FUNCTION_BLOCK Program_Assembled_Move_DUT

VAR_IN_OUT
    SD_SMD_IO: DUT_AMCI_Stepper;
END_VAR	

VAR_INPUT
	FB_Number_of_Segments: WORD; 
	
    FB_Segment_1_Distance: DINT;
    FB_Segment_1_Programmed_Speed: UDINT;
	FB_Segment_1_Acceleration: UINT;
	FB_Segment_1_Deceleration: UINT;
	
	FB_Segment_2_Distance: DINT;
    FB_Segment_2_Programmed_Speed: UDINT;
	FB_Segment_2_Acceleration: UINT;
	FB_Segment_2_Deceleration: UINT;
	
	FB_Segment_3_Distance: DINT;
    FB_Segment_3_Programmed_Speed: UDINT;
	FB_Segment_3_Acceleration: UINT;
	FB_Segment_3_Deceleration: UINT;
	
	FB_Segment_4_Distance: DINT;
    FB_Segment_4_Programmed_Speed: UDINT;
	FB_Segment_4_Acceleration: UINT;
	FB_Segment_4_Deceleration: UINT;
	
	FB_Segment_5_Distance: DINT;
    FB_Segment_5_Programmed_Speed: UDINT;
	FB_Segment_5_Acceleration: UINT;
	FB_Segment_5_Deceleration: UINT;
	
	FB_Segment_6_Distance: DINT;
    FB_Segment_6_Programmed_Speed: UDINT;
	FB_Segment_6_Acceleration: UINT;
	FB_Segment_6_Deceleration: UINT;
	
	FB_Segment_7_Distance: DINT;
    FB_Segment_7_Programmed_Speed: UDINT;
	FB_Segment_7_Acceleration: UINT;
	FB_Segment_7_Deceleration: UINT;
	
	FB_Segment_8_Distance: DINT;
    FB_Segment_8_Programmed_Speed: UDINT;
	FB_Segment_8_Acceleration: UINT;
	FB_Segment_8_Deceleration: UINT;
	
	FB_Segment_9_Distance: DINT;
    FB_Segment_9_Programmed_Speed: UDINT;
	FB_Segment_9_Acceleration: UINT;
	FB_Segment_9_Deceleration: UINT;
	
	FB_Segment_10_Distance: DINT;
    FB_Segment_10_Programmed_Speed: UDINT;
	FB_Segment_10_Acceleration: UINT;
	FB_Segment_10_Deceleration: UINT;
	
	FB_Segment_11_Distance: DINT;
    FB_Segment_11_Programmed_Speed: UDINT;
	FB_Segment_11_Acceleration: UINT;
	FB_Segment_11_Deceleration: UINT;
	
	FB_Segment_12_Distance: DINT;
    FB_Segment_12_Programmed_Speed: UDINT;
	FB_Segment_12_Acceleration: UINT;
	FB_Segment_12_Deceleration: UINT;
	
	FB_Segment_13_Distance: DINT;
    FB_Segment_13_Programmed_Speed: UDINT;
	FB_Segment_13_Acceleration: UINT;
	FB_Segment_13_Deceleration: UINT;
	
	FB_Segment_14_Distance: DINT;
    FB_Segment_14_Programmed_Speed: UDINT;
	FB_Segment_14_Acceleration: UINT;
	FB_Segment_14_Deceleration: UINT;
	
	FB_Segment_15_Distance: DINT;
    FB_Segment_15_Programmed_Speed: UDINT;
	FB_Segment_15_Acceleration: UINT;
	FB_Segment_15_Deceleration: UINT;
	
	FB_Segment_16_Distance: DINT;
    FB_Segment_16_Programmed_Speed: UDINT;
	FB_Segment_16_Acceleration: UINT;
	FB_Segment_16_Deceleration: UINT;
	
END_VAR

VAR_OUTPUT
	Enable: BOOL :=FALSE;
	Error: BOOL :=TRUE;
	Assembled_Move_Programmed: BOOL;
	
END_VAR

VAR	
	I_Command_Word_1: UINT;
	Assembled_Move_counter: ctu;
	Assembled_Move_counter_CV: DINT;
	Assembled_move_counter_PV: WORD;
	Assembled_Move_counter_DN: BOOL;
	Assembled_move_counter_reset: BOOL;
	
	
	
END_VAR
VAR // added by the converter: edge detectors and wires of the graphical bodies
    _w1, _w2, _w3, _w4, _w5, _w6, _w7, _w8, _w9, _w10, _w11, _w12, _w13, _w14, _w15, _w16, _w17, _w18, _w19 : BOOL;
END_VAR

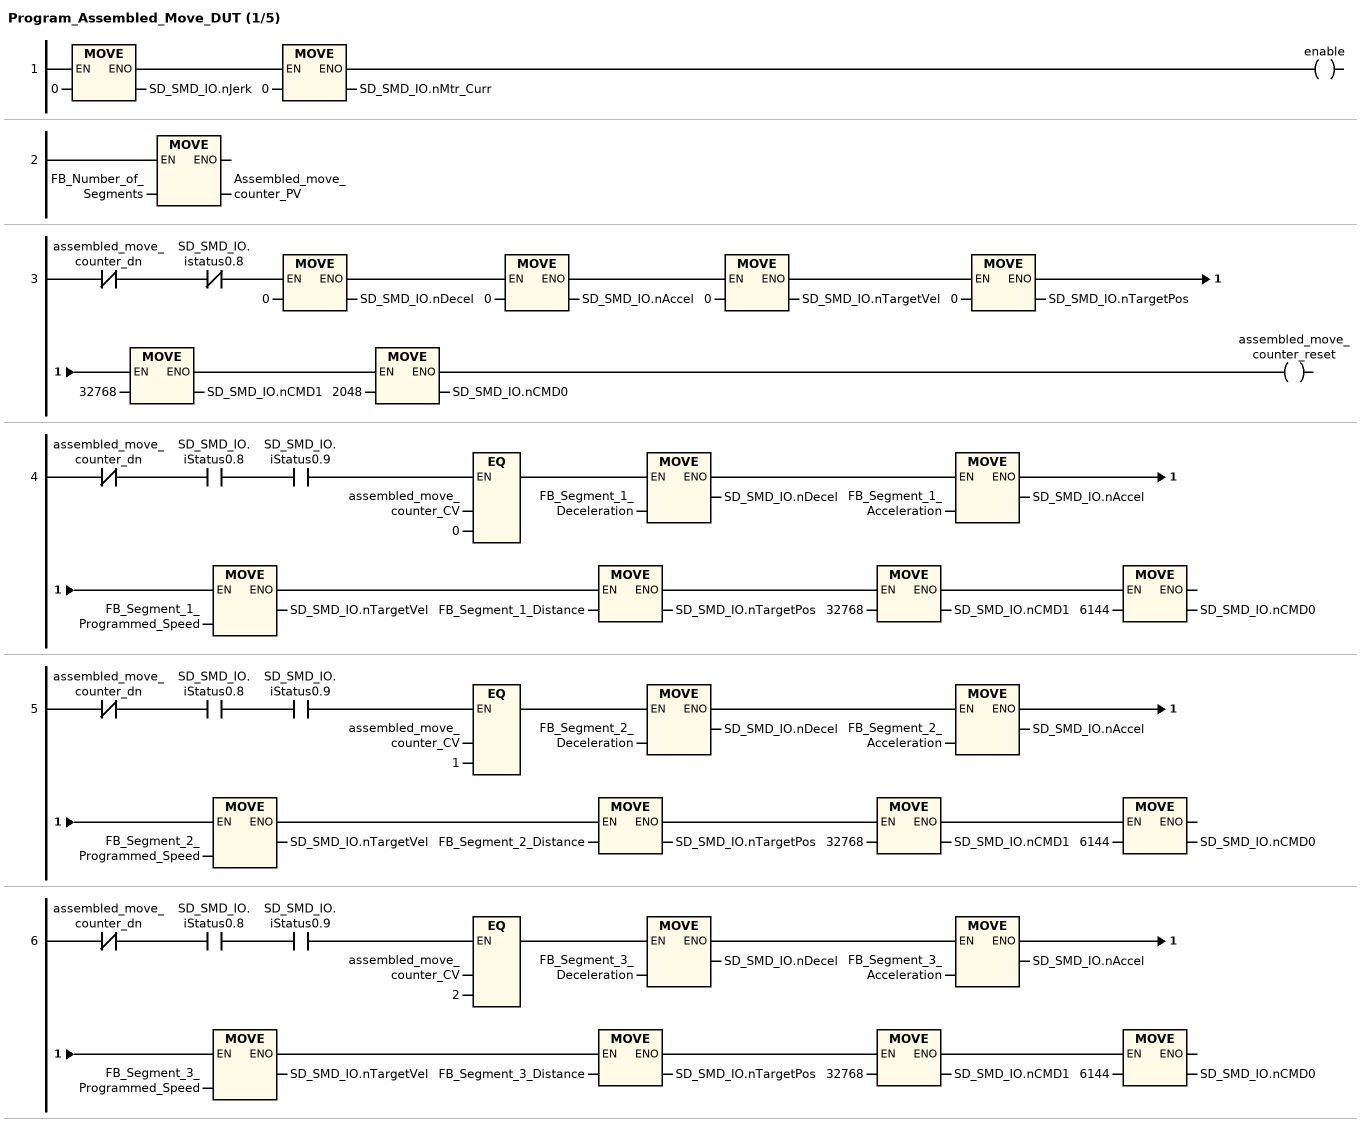
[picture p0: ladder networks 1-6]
// NETWORK 1
SD_SMD_IO.nJerk := 0;
SD_SMD_IO.nMtr_Curr := 0;
enable := TRUE;

// NETWORK 2
Assembled_move_counter_PV := FB_Number_of_Segments;

// NETWORK 3
_w1 := NOT assembled_move_counter_dn AND NOT SD_SMD_IO.istatus0.8;
IF _w1 THEN SD_SMD_IO.nDecel := 0; END_IF
IF _w1 THEN SD_SMD_IO.nAccel := 0; END_IF
IF _w1 THEN SD_SMD_IO.nTargetVel := 0; END_IF
IF _w1 THEN SD_SMD_IO.nTargetPos := 0; END_IF
IF _w1 THEN SD_SMD_IO.nCMD1 := 32768; END_IF
IF _w1 THEN SD_SMD_IO.nCMD0 := 2048; END_IF
assembled_move_counter_reset := _w1;

// NETWORK 4
_w2 := NOT assembled_move_counter_dn AND SD_SMD_IO.iStatus0.8 AND SD_SMD_IO.iStatus0.9 AND assembled_move_counter_CV = 0;
IF _w2 THEN SD_SMD_IO.nDecel := FB_Segment_1_Deceleration; END_IF
IF _w2 THEN SD_SMD_IO.nAccel := FB_Segment_1_Acceleration; END_IF
IF _w2 THEN SD_SMD_IO.nTargetVel := FB_Segment_1_Programmed_Speed; END_IF
IF _w2 THEN SD_SMD_IO.nTargetPos := FB_Segment_1_Distance; END_IF
IF _w2 THEN SD_SMD_IO.nCMD1 := 32768; END_IF
IF _w2 THEN SD_SMD_IO.nCMD0 := 6144; END_IF

// NETWORK 5
_w3 := NOT assembled_move_counter_dn AND SD_SMD_IO.iStatus0.8 AND SD_SMD_IO.iStatus0.9 AND assembled_move_counter_CV = 1;
IF _w3 THEN SD_SMD_IO.nDecel := FB_Segment_2_Deceleration; END_IF
IF _w3 THEN SD_SMD_IO.nAccel := FB_Segment_2_Acceleration; END_IF
IF _w3 THEN SD_SMD_IO.nTargetVel := FB_Segment_2_Programmed_Speed; END_IF
IF _w3 THEN SD_SMD_IO.nTargetPos := FB_Segment_2_Distance; END_IF
IF _w3 THEN SD_SMD_IO.nCMD1 := 32768; END_IF
IF _w3 THEN SD_SMD_IO.nCMD0 := 6144; END_IF

// NETWORK 6
_w4 := NOT assembled_move_counter_dn AND SD_SMD_IO.iStatus0.8 AND SD_SMD_IO.iStatus0.9 AND assembled_move_counter_CV = 2;
IF _w4 THEN SD_SMD_IO.nDecel := FB_Segment_3_Deceleration; END_IF
IF _w4 THEN SD_SMD_IO.nAccel := FB_Segment_3_Acceleration; END_IF
IF _w4 THEN SD_SMD_IO.nTargetVel := FB_Segment_3_Programmed_Speed; END_IF
IF _w4 THEN SD_SMD_IO.nTargetPos := FB_Segment_3_Distance; END_IF
IF _w4 THEN SD_SMD_IO.nCMD1 := 32768; END_IF
IF _w4 THEN SD_SMD_IO.nCMD0 := 6144; END_IF

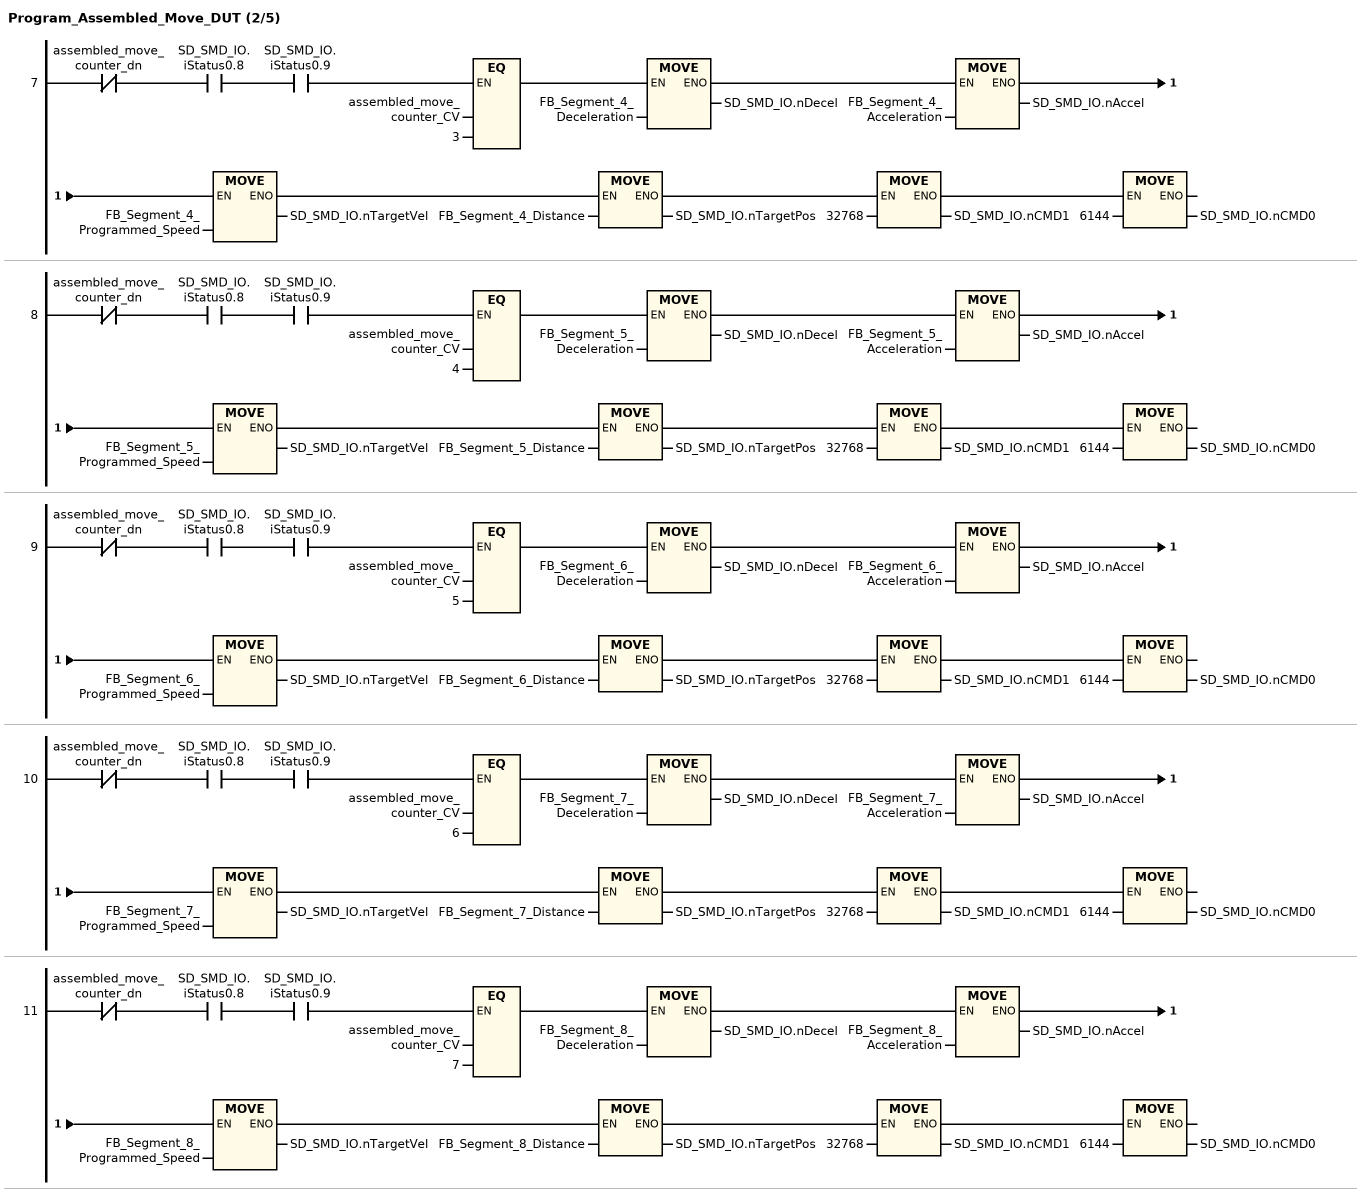
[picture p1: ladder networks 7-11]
// NETWORK 7
_w5 := NOT assembled_move_counter_dn AND SD_SMD_IO.iStatus0.8 AND SD_SMD_IO.iStatus0.9 AND assembled_move_counter_CV = 3;
IF _w5 THEN SD_SMD_IO.nDecel := FB_Segment_4_Deceleration; END_IF
IF _w5 THEN SD_SMD_IO.nAccel := FB_Segment_4_Acceleration; END_IF
IF _w5 THEN SD_SMD_IO.nTargetVel := FB_Segment_4_Programmed_Speed; END_IF
IF _w5 THEN SD_SMD_IO.nTargetPos := FB_Segment_4_Distance; END_IF
IF _w5 THEN SD_SMD_IO.nCMD1 := 32768; END_IF
IF _w5 THEN SD_SMD_IO.nCMD0 := 6144; END_IF

// NETWORK 8
_w6 := NOT assembled_move_counter_dn AND SD_SMD_IO.iStatus0.8 AND SD_SMD_IO.iStatus0.9 AND assembled_move_counter_CV = 4;
IF _w6 THEN SD_SMD_IO.nDecel := FB_Segment_5_Deceleration; END_IF
IF _w6 THEN SD_SMD_IO.nAccel := FB_Segment_5_Acceleration; END_IF
IF _w6 THEN SD_SMD_IO.nTargetVel := FB_Segment_5_Programmed_Speed; END_IF
IF _w6 THEN SD_SMD_IO.nTargetPos := FB_Segment_5_Distance; END_IF
IF _w6 THEN SD_SMD_IO.nCMD1 := 32768; END_IF
IF _w6 THEN SD_SMD_IO.nCMD0 := 6144; END_IF

// NETWORK 9
_w7 := NOT assembled_move_counter_dn AND SD_SMD_IO.iStatus0.8 AND SD_SMD_IO.iStatus0.9 AND assembled_move_counter_CV = 5;
IF _w7 THEN SD_SMD_IO.nDecel := FB_Segment_6_Deceleration; END_IF
IF _w7 THEN SD_SMD_IO.nAccel := FB_Segment_6_Acceleration; END_IF
IF _w7 THEN SD_SMD_IO.nTargetVel := FB_Segment_6_Programmed_Speed; END_IF
IF _w7 THEN SD_SMD_IO.nTargetPos := FB_Segment_6_Distance; END_IF
IF _w7 THEN SD_SMD_IO.nCMD1 := 32768; END_IF
IF _w7 THEN SD_SMD_IO.nCMD0 := 6144; END_IF

// NETWORK 10
_w8 := NOT assembled_move_counter_dn AND SD_SMD_IO.iStatus0.8 AND SD_SMD_IO.iStatus0.9 AND assembled_move_counter_CV = 6;
IF _w8 THEN SD_SMD_IO.nDecel := FB_Segment_7_Deceleration; END_IF
IF _w8 THEN SD_SMD_IO.nAccel := FB_Segment_7_Acceleration; END_IF
IF _w8 THEN SD_SMD_IO.nTargetVel := FB_Segment_7_Programmed_Speed; END_IF
IF _w8 THEN SD_SMD_IO.nTargetPos := FB_Segment_7_Distance; END_IF
IF _w8 THEN SD_SMD_IO.nCMD1 := 32768; END_IF
IF _w8 THEN SD_SMD_IO.nCMD0 := 6144; END_IF

// NETWORK 11
_w9 := NOT assembled_move_counter_dn AND SD_SMD_IO.iStatus0.8 AND SD_SMD_IO.iStatus0.9 AND assembled_move_counter_CV = 7;
IF _w9 THEN SD_SMD_IO.nDecel := FB_Segment_8_Deceleration; END_IF
IF _w9 THEN SD_SMD_IO.nAccel := FB_Segment_8_Acceleration; END_IF
IF _w9 THEN SD_SMD_IO.nTargetVel := FB_Segment_8_Programmed_Speed; END_IF
IF _w9 THEN SD_SMD_IO.nTargetPos := FB_Segment_8_Distance; END_IF
IF _w9 THEN SD_SMD_IO.nCMD1 := 32768; END_IF
IF _w9 THEN SD_SMD_IO.nCMD0 := 6144; END_IF

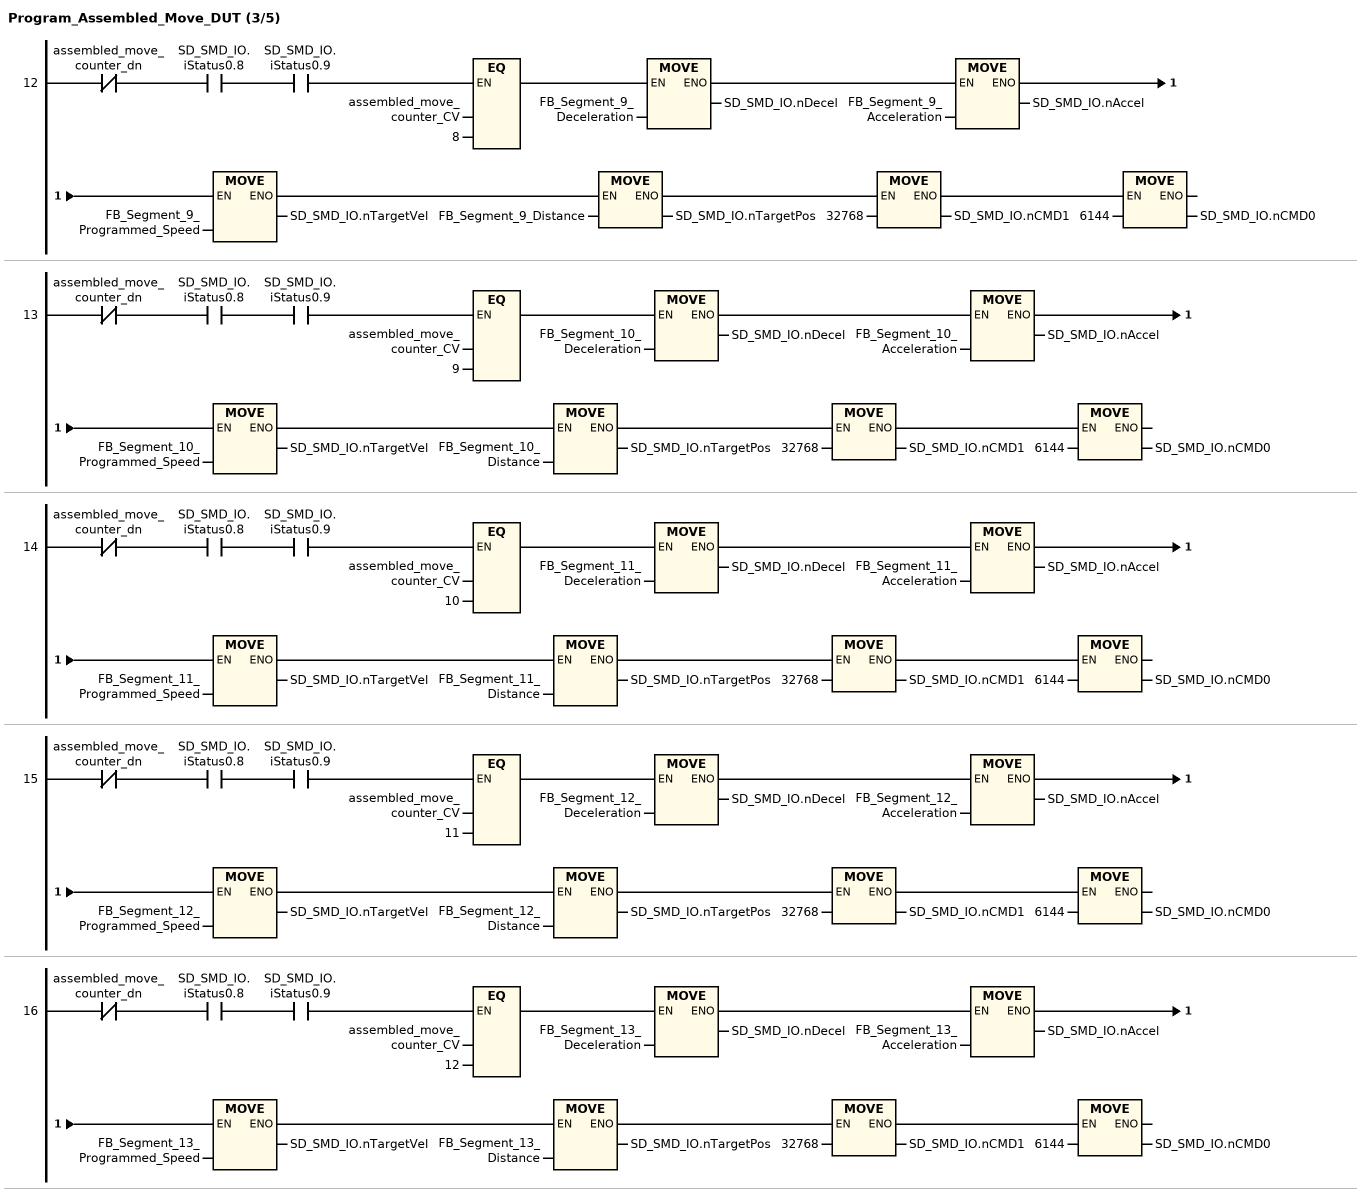
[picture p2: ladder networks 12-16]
// NETWORK 12
_w10 := NOT assembled_move_counter_dn AND SD_SMD_IO.iStatus0.8 AND SD_SMD_IO.iStatus0.9 AND assembled_move_counter_CV = 8;
IF _w10 THEN SD_SMD_IO.nDecel := FB_Segment_9_Deceleration; END_IF
IF _w10 THEN SD_SMD_IO.nAccel := FB_Segment_9_Acceleration; END_IF
IF _w10 THEN SD_SMD_IO.nTargetVel := FB_Segment_9_Programmed_Speed; END_IF
IF _w10 THEN SD_SMD_IO.nTargetPos := FB_Segment_9_Distance; END_IF
IF _w10 THEN SD_SMD_IO.nCMD1 := 32768; END_IF
IF _w10 THEN SD_SMD_IO.nCMD0 := 6144; END_IF

// NETWORK 13
_w11 := NOT assembled_move_counter_dn AND SD_SMD_IO.iStatus0.8 AND SD_SMD_IO.iStatus0.9 AND assembled_move_counter_CV = 9;
IF _w11 THEN SD_SMD_IO.nDecel := FB_Segment_10_Deceleration; END_IF
IF _w11 THEN SD_SMD_IO.nAccel := FB_Segment_10_Acceleration; END_IF
IF _w11 THEN SD_SMD_IO.nTargetVel := FB_Segment_10_Programmed_Speed; END_IF
IF _w11 THEN SD_SMD_IO.nTargetPos := FB_Segment_10_Distance; END_IF
IF _w11 THEN SD_SMD_IO.nCMD1 := 32768; END_IF
IF _w11 THEN SD_SMD_IO.nCMD0 := 6144; END_IF

// NETWORK 14
_w12 := NOT assembled_move_counter_dn AND SD_SMD_IO.iStatus0.8 AND SD_SMD_IO.iStatus0.9 AND assembled_move_counter_CV = 10;
IF _w12 THEN SD_SMD_IO.nDecel := FB_Segment_11_Deceleration; END_IF
IF _w12 THEN SD_SMD_IO.nAccel := FB_Segment_11_Acceleration; END_IF
IF _w12 THEN SD_SMD_IO.nTargetVel := FB_Segment_11_Programmed_Speed; END_IF
IF _w12 THEN SD_SMD_IO.nTargetPos := FB_Segment_11_Distance; END_IF
IF _w12 THEN SD_SMD_IO.nCMD1 := 32768; END_IF
IF _w12 THEN SD_SMD_IO.nCMD0 := 6144; END_IF

// NETWORK 15
_w13 := NOT assembled_move_counter_dn AND SD_SMD_IO.iStatus0.8 AND SD_SMD_IO.iStatus0.9 AND assembled_move_counter_CV = 11;
IF _w13 THEN SD_SMD_IO.nDecel := FB_Segment_12_Deceleration; END_IF
IF _w13 THEN SD_SMD_IO.nAccel := FB_Segment_12_Acceleration; END_IF
IF _w13 THEN SD_SMD_IO.nTargetVel := FB_Segment_12_Programmed_Speed; END_IF
IF _w13 THEN SD_SMD_IO.nTargetPos := FB_Segment_12_Distance; END_IF
IF _w13 THEN SD_SMD_IO.nCMD1 := 32768; END_IF
IF _w13 THEN SD_SMD_IO.nCMD0 := 6144; END_IF

// NETWORK 16
_w14 := NOT assembled_move_counter_dn AND SD_SMD_IO.iStatus0.8 AND SD_SMD_IO.iStatus0.9 AND assembled_move_counter_CV = 12;
IF _w14 THEN SD_SMD_IO.nDecel := FB_Segment_13_Deceleration; END_IF
IF _w14 THEN SD_SMD_IO.nAccel := FB_Segment_13_Acceleration; END_IF
IF _w14 THEN SD_SMD_IO.nTargetVel := FB_Segment_13_Programmed_Speed; END_IF
IF _w14 THEN SD_SMD_IO.nTargetPos := FB_Segment_13_Distance; END_IF
IF _w14 THEN SD_SMD_IO.nCMD1 := 32768; END_IF
IF _w14 THEN SD_SMD_IO.nCMD0 := 6144; END_IF

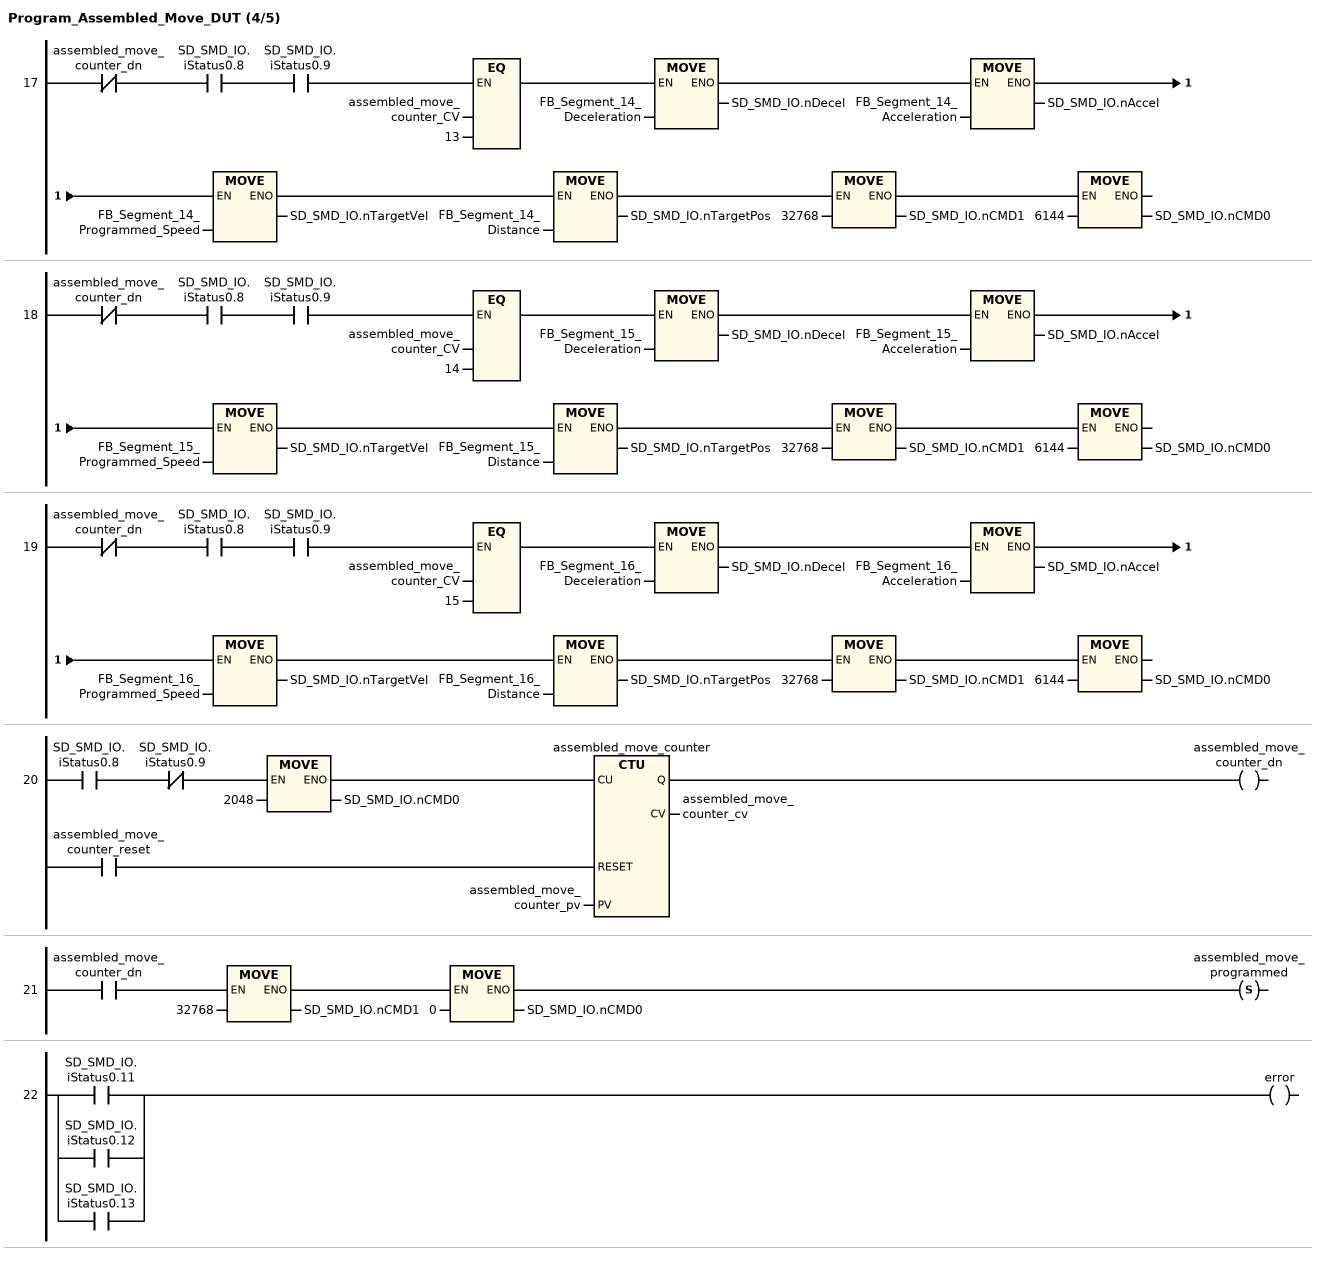
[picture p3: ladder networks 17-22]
// NETWORK 17
_w15 := NOT assembled_move_counter_dn AND SD_SMD_IO.iStatus0.8 AND SD_SMD_IO.iStatus0.9 AND assembled_move_counter_CV = 13;
IF _w15 THEN SD_SMD_IO.nDecel := FB_Segment_14_Deceleration; END_IF
IF _w15 THEN SD_SMD_IO.nAccel := FB_Segment_14_Acceleration; END_IF
IF _w15 THEN SD_SMD_IO.nTargetVel := FB_Segment_14_Programmed_Speed; END_IF
IF _w15 THEN SD_SMD_IO.nTargetPos := FB_Segment_14_Distance; END_IF
IF _w15 THEN SD_SMD_IO.nCMD1 := 32768; END_IF
IF _w15 THEN SD_SMD_IO.nCMD0 := 6144; END_IF

// NETWORK 18
_w16 := NOT assembled_move_counter_dn AND SD_SMD_IO.iStatus0.8 AND SD_SMD_IO.iStatus0.9 AND assembled_move_counter_CV = 14;
IF _w16 THEN SD_SMD_IO.nDecel := FB_Segment_15_Deceleration; END_IF
IF _w16 THEN SD_SMD_IO.nAccel := FB_Segment_15_Acceleration; END_IF
IF _w16 THEN SD_SMD_IO.nTargetVel := FB_Segment_15_Programmed_Speed; END_IF
IF _w16 THEN SD_SMD_IO.nTargetPos := FB_Segment_15_Distance; END_IF
IF _w16 THEN SD_SMD_IO.nCMD1 := 32768; END_IF
IF _w16 THEN SD_SMD_IO.nCMD0 := 6144; END_IF

// NETWORK 19
_w17 := NOT assembled_move_counter_dn AND SD_SMD_IO.iStatus0.8 AND SD_SMD_IO.iStatus0.9 AND assembled_move_counter_CV = 15;
IF _w17 THEN SD_SMD_IO.nDecel := FB_Segment_16_Deceleration; END_IF
IF _w17 THEN SD_SMD_IO.nAccel := FB_Segment_16_Acceleration; END_IF
IF _w17 THEN SD_SMD_IO.nTargetVel := FB_Segment_16_Programmed_Speed; END_IF
IF _w17 THEN SD_SMD_IO.nTargetPos := FB_Segment_16_Distance; END_IF
IF _w17 THEN SD_SMD_IO.nCMD1 := 32768; END_IF
IF _w17 THEN SD_SMD_IO.nCMD0 := 6144; END_IF

// NETWORK 20
_w18 := SD_SMD_IO.iStatus0.8 AND NOT SD_SMD_IO.iStatus0.9;
IF _w18 THEN SD_SMD_IO.nCMD0 := 2048; END_IF
assembled_move_counter(
    CU := _w18,
    RESET := assembled_move_counter_reset,
    PV := assembled_move_counter_pv,
    CV => assembled_move_counter_cv); // CTU
assembled_move_counter_dn := assembled_move_counter.Q;

// NETWORK 21
_w19 := assembled_move_counter_dn;
IF _w19 THEN SD_SMD_IO.nCMD1 := 32768; END_IF
IF _w19 THEN SD_SMD_IO.nCMD0 := 0; END_IF
assembled_move_programmed S= _w19;

// NETWORK 22
error := SD_SMD_IO.iStatus0.11 OR SD_SMD_IO.iStatus0.12 OR SD_SMD_IO.iStatus0.13;

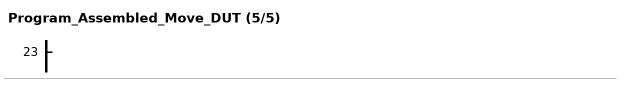
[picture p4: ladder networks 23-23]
// NETWORK 23

END_FUNCTION_BLOCK
